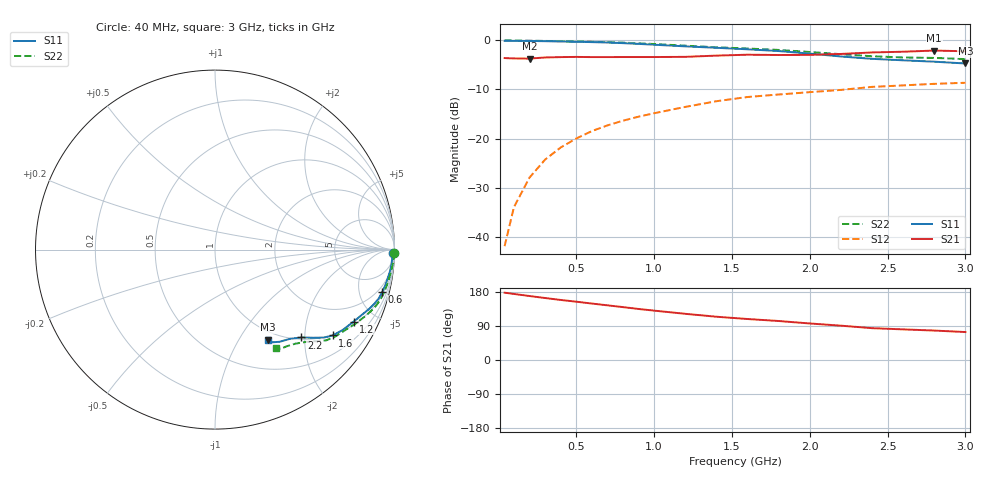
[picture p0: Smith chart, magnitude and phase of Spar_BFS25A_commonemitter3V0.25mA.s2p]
! Filename:  BFS25AG.S2P  Version:  4.0
! NXP part #: BFS25A  Date: Jun 1994
! Bias condition: Vce=3V, Ic=0.25mA
#  MHz  S  MA  R  50
! Freq  S11  S21  S12  S22  !GUM [dB]
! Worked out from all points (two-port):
!   21 points, 40 MHz to 3 GHz, reference 50 ohm
!   highest |S21| = -2.07 dB at 2.8 GHz (marker M1); lowest = -3.7 dB at 200 MHz (marker M2)
!   |S21| within 3 dB of the highest: start of sweep to end of sweep
!   lowest |S11| = -4.7 dB at 3 GHz (marker M3), VSWR 3.78, Z = 44 - j66.9 ohm
!   |S11| at or under -10 dB: nowhere
!   |S22| runs from -3.8 to 0.0 dB; largest |S21 - S12| = 0.67
!   S11 on the Smith chart (normalised r, x): 40 MHz: open; 600 MHz: 1.25, -7.77; 1.2 GHz: 1.14, -3.76; 1.6 GHz: 0.98, -2.76; 2.2 GHz: 1.04, -1.92; 3 GHz: 0.88, -1.34
40  0.99 -1.0  0.661 177.6  0.008 88.3  0.999 -1.0
100  0.989 -2.3  0.655 174.3  0.02 85.9  0.998 -2.5
200  0.987 -4.7  0.653 168.8  0.04 83.7  0.993 -4.9
300  0.982 -7.2  0.67 163.6  0.061 81.3  0.988 -7.5
400  0.975 -9.7  0.676 158.5  0.081 79.2  0.982 -10.1
500  0.969 -12.0  0.679 153.9  0.1 77.3  0.976 -12.6
600  0.961 -14.3  0.676 149.0  0.119 75.4  0.969 -15.1
700  0.952 -16.6  0.676 144.3  0.136 73.5  0.96 -17.4
800  0.938 -18.7  0.677 139.6  0.152 71.5  0.949 -19.4
900  0.922 -20.8  0.677 134.7  0.167 69.2  0.934 -21.5
1000  0.904 -22.9  0.677 130.3  0.181 66.9  0.919 -23.5
1200  0.87 -27.5  0.68 121.9  0.21 62.2  0.884 -27.9
1400  0.841 -32.1  0.7 114.2  0.24 58.5  0.851 -32.0
1600  0.812 -36.1  0.715 108.2  0.265 55.0  0.827 -35.8
1800  0.779 -39.0  0.71 102.9  0.281 52.9  0.8 -39.2
2000  0.734 -42.0  0.712 96.4  0.297 49.7  0.762 -42.0
2200  0.686 -45.5  0.728 90.6  0.313 47.0  0.724 -45.2
2400  0.649 -50.0  0.754 84.0  0.336 43.7  0.69 -49.4
2600  0.627 -55.0  0.767 80.8  0.348 41.1  0.67 -53.6
2800  0.607 -58.3  0.788 77.7  0.361 40.5  0.663 -56.5
3000  0.582 -59.7  0.775 73.8  0.37 38.9  0.646 -58.3
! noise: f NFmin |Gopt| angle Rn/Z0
500  1.6  0.927  2  3.7
1000  1.8  0.903  7  3.4
2000  2  0.694  29  2
